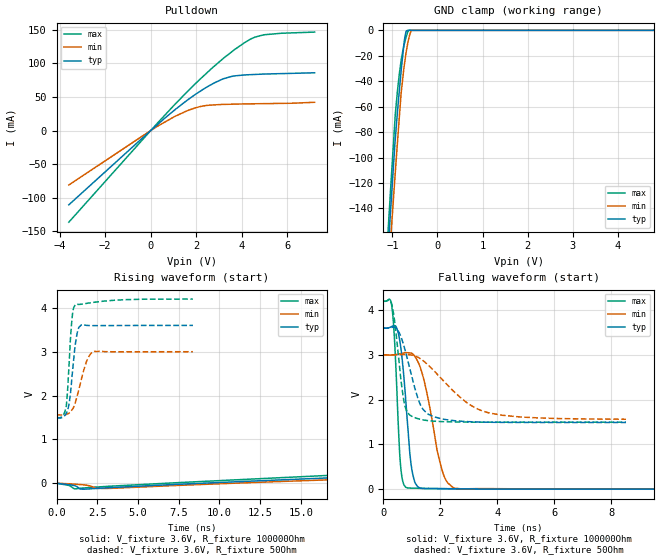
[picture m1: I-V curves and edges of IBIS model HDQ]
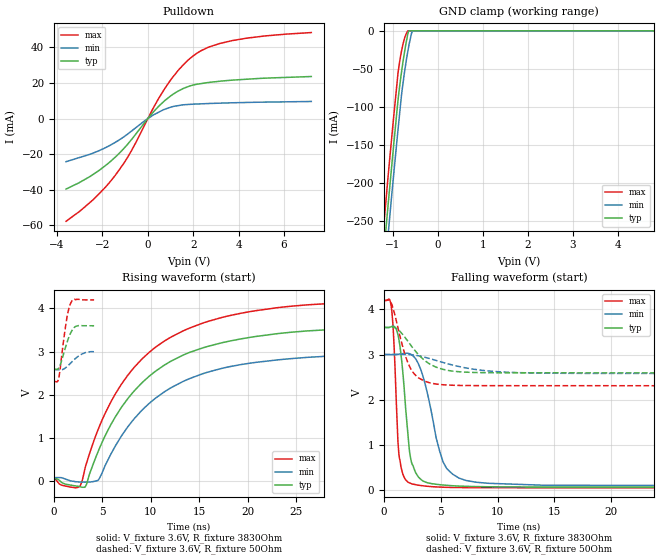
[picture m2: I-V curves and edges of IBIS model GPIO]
|Texas Instruments Incorporated
|Single-Cell Li-Ion and Li-Pol Battery Gas Gauge IC for Portable Applications
|   (bqJunior)
| Marketing part#   Digital Voltage Range   Package-type   #pins
| BQ27000DRKR   2.6 to 4.5V   VSON   10
| BQ27000DRKRG4   2.6 to 4.5V   VSON   10
[IBIS Ver]   3.2
[File name]   bq27000.ibs
|SIMDE Ver   V2.0 - 201002 - RHL4 - Build 372
[File Rev]   1.5
[Date]   08/18/2010
[Source]
|   Texas Instruments Incorporated.
|   Analog-eLab Design Center, HPA
|   12500 TI Blvd
|   Dallas, TX -75243
|   e-mail: elab_ibis@list.ti.com
| Model generated from simulations in TISPICE
[Notes]   Revision History:
|   Rev 1.0: 06/16/2010
|   - Initial version of the model
|   - Model names with a trailing 3p3pv contains the model for
|   3.3V [2.6V and 4.2V]. Model names with trailing 4p4v contains
|   the model for 4.4V [4.3V and 4.5V] operation.Model names with
|   trailing 3p5v contains the model for 3.55V [2.6 and 4.5V]
|   operation.
|   Rev 1.1: 07/02/2010
|   - Model generated from simulations in TISPICE
|   - Model matched to SPICE simulation
|   - Updated the ibis file with data sheet title and package
|   details
|   - While calculating R_pkg, L_pkg and C_pkg ignored values
|   corresponding to power and ground pins
|   - Added package details beside [Package]
|   - Updated the buffer ibis models with correct voltage ranges
|   - Model names with a trailing 3p6v contains the model for
|   3.6V [3.0V and 4.2V].
|   - C_comp although listed in numerical order of value are obtained
|   from varying PVT conditions. For PVT conditions for each specific
|   value refer the buffer description under respective [Model]. IBIS
|   model user is responsible for using appropriate C_comp to simulate
|   for Signal Integrity.
|*   EXCEPTION:   *
|*   - input_mode1_3p6v,input_mode2_3p6v and input_mode4_3p6v there will*
|*   be a leakage current in the clamp I-V table because of the   *
|*   pulldown on pad.   *
|   Rev 1.2: 07/13/2010
|   - IBIS models generated with updated temperature range(-20/25/70)
|   - Updated the package details.
|   - Removed input IBIS models with weak pulldown to pad.
|*   EXCEPTION:   *
|*   - input_mode4_3p6v there will be a leakage current in the clamp I-V*
|*   table because of the pulldown on pad.   *
|   Rev 1.3: 07/28/2010
|   - Changed open_drain model to io_open_drain
|   - Updated the package details.
|   - Corrected over voltage entries for INPUT buffer power clamp and
|   ground clamp tables.
|*   EXCEPTION:   *
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[Disclaimer]
| This model is designed as an aid for customers of Texas Instruments.
| TI and its licensors and suppliers make no warranties, either expressed
| or implied, with respect to this  model, including the warranties of
| merchantability or fitness for a particular purpose. The model is
| provided solely on an "as is" basis. The entire risk as to its quality
| and performance is with the customer.
[Copyright]
|(C) Copyright 2010 Texas Instruments Incorporated.All rights reserved.
|   BQ27000
[Component]   BQ27000
[Manufacturer]  TI
[Package]   | 10 VSON - DRK package
|   typ   min   max
R_pkg   0.049698   0.04509   0.0584
L_pkg   0.910128nH   0.82212nH   1.09342nH
C_pkg   0.140814pF   0.12909pF   0.15381pF
[Pin]  signal_name model_name   R_pin   L_pin   C_pin
1   RBI   TERM   0.05840   1.09342nH   0.14472pF
2   VCC   POWER   0.05274   0.97555nH   0.15314pF
3   VSS   GND   0.04627   0.84523nH   0.14454pF
4   D/C   TERM   0.04509   0.82212nH   0.14082pF
5   HDQ   HDQ   0.04667   0.85344nH   0.12909pF
6   BAT   TERM   0.04824   0.87702nH   0.13320pF
7   SRN   TERM   0.04798   0.87136nH   0.14749pF
8   SRP   TERM   0.05430   1.00150nH   0.15381pF
9   GPIO   GPIO   0.04775   0.86672nH   0.14403pF
10   PGM   TERM   0.04915   0.89544nH   0.13335pF
11   VSS   GND   0.00002   0.05199nH   0.50818pF
|   TERM Model
[Model] TERM
Model_type Terminator
C_comp   0   0   0
| variable   typ   min   max
[Voltage Range]   3.6   3   4.2
[POWER Clamp Reference]  3.6   3   4.2
[GND Clamp Reference]   0.0V   0.0V   0.0V
|Operating Temperature
[Temperature Range]   25   70   -20
| Models and submodels in the file (3): HDQ (I/O_open_drain), GPIO (I/O_open_drain), TERM (Terminator)
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|   HDQ Model
[Model]   HDQ
Model_type   I/O_open_drain
Polarity   Inverting
Enable   Active-Low
Vinl = 0.7
Vinh = 1.5
Vmeas = 1.8
Vref = 3.6
Cref = 5pF
Rref = 100000
|   typ   min   max
|   (nom PVT)   (Fast PVT)   (Slow PVT)
|Average
C_comp   2.068e-12   1.732e-12   2.876e-12
|OFF state: BUFFER in HIGH IMPEDANCE
|C_comp   1.649e-12   1.632e-12   1.682e-12
|ON state : BUFFER OUTPUT TURNED LOW
|C_comp   2.487e-12   1.832e-12   4.071e-12
[Voltage Range]   3.6   3   4.2
|Ambient Temperature   25   70   -20
|Junction Temperature
[Temperature Range]   25   70   -20
[Pullup Reference]   3.6   3   4.2
[Pulldown Reference]   0   0   0
[Power Clamp Reference]   3.6   3   4.2
[GND Clamp Reference]   0   0   0
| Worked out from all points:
|   slope of the pulldown table from 0 to 0.54 V, typ, clamps not added: 33.7 ohm
|   GND clamp passes 1 mA (typ) near -0.70 V on its own axis
|   falling waveform, V_fixture 3.6V, R_fixture 100000Ohm: 20-80 % time 279ps typ, 549ps min, 180ps max; typ from 3.6 V to 0.001 V
|   rising waveform, V_fixture 3.6V, R_fixture 100000Ohm: 20-80 % time 225ns typ, 230ns min, 223ns max; typ from 0.001 V to 3.6 V
|   falling waveform, V_fixture 3.6V, R_fixture 50Ohm: 20-80 % time 551ps typ, 1.46ns min, 291ps max; typ from 3.6 V to 1.49 V
|   rising waveform, V_fixture 3.6V, R_fixture 50Ohm: 20-80 % time 350ps typ, 624ps min, 265ps max; typ from 1.49 V to 3.6 V
[Pulldown]
|   Voltage   I(typ)   I(min)   I(max)
-3.6V     -110.5mA   -81.05mA   -136.3mA
0V        0A         0A         0A
1.035V    30.07mA    20.52mA    37.86mA
1.674V    46.81mA    30.34mA    59.98mA
2.223V    59.47mA    35.97mA    78.03mA
2.794V    70.82mA    38.11mA    95.68mA
3.146V    76.31mA    38.77mA    106mA
3.683V    81.19mA    39.21mA    120.3mA
4.38V     83.04mA    39.68mA    135.8mA
4.582V    83.35mA    39.77mA    138.9mA
4.968V    83.94mA    39.95mA    142.3mA
7.2V      85.83mA    41.98mA    146.3mA
[GND Clamp]
|   Voltage   I(typ)   I(min)   I(max)
-3.6V     -1.773A    -1.701A    -1.839A
-1.143V   -199.5mA   -220.7mA   -185.7mA
-1.055V   -149.5mA   -172.9mA   -133.3mA
-1.023V   -131.9mA   -155.7mA   -115.1mA
-937.2mV  -85.84mA   -112.2mA   -66.69mA
-891mV    -65.5mA    -89.46mA   -48.68mA
-807mV    -32.17mA   -49.63mA   -23.81mA
-730.8mV  -7.013mA   -26.14mA   -10.08mA
-694.8mV  -545.6uA   -17.14mA   -5.281mA
-660mV    0A         -10.17mA   -1.416mA
-576mV    0A         0A         0A
7.2V      0A         0A         0A
[POWER Clamp]
|   Voltage   I(typ)   I(min)   I(max)
-3.6V     0A         0A         0A
7.2V      0A         0A         0A
[Ramp]
R_load = 100000
|   typ   min   max
dV/dt_r   2.15645/2.25529e-07   1.79638/2.30137e-07   2.51628/2.23208e-07
dV/dt_f   2.15929/2.80954e-10   1.79917/5.49564e-10   2.51932/1.84623e-10
[Falling Waveform]
V_fixture = 3.6V
V_fixture_min = 3V
V_fixture_max = 4.2V
R_fixture = 100000Ohm
|   Time   V(typ)   V(min)   V(max)
0s        3.6V       3V         4.2V
300ps     3.638V     2.999V     4.067V
400ps     3.65V      3.005V     3.229V
600ps     3.218V     3.028V     550.5mV
875ps     1.242V     3.048V     25.56mV
1ns       440.2mV    3.037V     23.89mV
1.2ns     59.77mV    2.864V     21.87mV
2.1ns     14.42mV    346.7mV    8.533mV
2.55ns    9.999mV    16.73mV    6.274mV
40ns      1.209mV    1.432mV    1.127mV
[Rising Waveform]
V_fixture = 3.6V
V_fixture_min = 3V
V_fixture_max = 4.2V
R_fixture = 100000Ohm
|   Time   V(typ)   V(min)   V(max)
0s        1.177mV    1.371mV    1.116mV
1.7ns     -132.9mV   -36.04mV   -105.1mV
3.25ns    -98.77mV   -115.3mV   -66.45mV
82ns      1.089V     882.5mV    1.301V
167.2ns   2.074V     1.696V     2.456V
241.1ns   2.651V     2.18V      3.123V
325.4ns   3.063V     2.528V     3.594V
423.2ns   3.326V     2.756V     3.894V
548.5ns   3.486V     2.896V     4.074V
1us       3.595V     2.995V     4.195V
[Falling Waveform]
V_fixture = 3.6V
V_fixture_min = 3V
V_fixture_max = 4.2V
R_fixture = 50Ohm
|   Time   V(typ)   V(min)   V(max)
0s        3.6V       3V         4.2V
300ps     3.616V     3.001V     4.114V
500ps     3.559V     3.006V     3.15V
725ps     3.19V      3.009V     1.953V
1.05ns    2.391V     2.991V     1.612V
1.3ns     1.886V     2.914V     1.561V
1.6ns     1.667V     2.757V     1.53V
2.9ns     1.512V     1.949V     1.5V
3.6ns     1.497V     1.724V     1.499V
8.525ns   1.491V     1.563V     1.498V
[Rising Waveform]
V_fixture = 3.6V
V_fixture_min = 3V
V_fixture_max = 4.2V
R_fixture = 50Ohm
|   Time   V(typ)   V(min)   V(max)
0s        1.49V      1.56V      1.498V
375ps     1.504V     1.556V     1.538V
600ps     1.599V     1.57V      1.768V
775ps     1.828V     1.603V     2.736V
925ps     2.322V     1.661V     3.641V
1.15ns    3.151V     1.837V     4.069V
1.4ns     3.567V     2.179V     4.078V
1.825ns   3.601V     2.759V     4.1V
2.25ns    3.594V     3V         4.123V
8.375ns   3.599V     2.999V     4.199V
|   GPIO Model
[Model]   GPIO
Model_type   I/O_open_drain
Polarity   Non-Inverting
Enable   Active-Low
Vinl = 0.7
Vinh = 1.5
Vmeas = 1.8
Vref = 3.6
Cref = 5pF
Rref = 3830
|   typ   min   max
|   (nom PVT)   (Fast PVT)   (Slow PVT)
|Average
C_comp   3.532e-12   2.936e-12   3.781e-12
|ON state : BUFFER OUTPUT TURNED LOW
|C_comp   5.491e-12   4.260e-12   6.024e-12
|OFF state: BUFFER in HIGH IMPEDANCE
|C_comp   1.574e-12   1.613e-12   1.538e-12
[Voltage Range]   3.6   3   4.2
|Ambient Temperature   25   70   -20
|Junction Temperature
[Temperature Range]   25   70   -20
[Pullup Reference]   3.6   3   4.2
[Pulldown Reference]   0   0   0
[Power Clamp Reference]   3.6   3   4.2
[GND Clamp Reference]   0   0   0
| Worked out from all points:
|   slope of the pulldown table from 0 to 0.54 V, typ, clamps not added: 70.8 ohm
|   GND clamp passes 1 mA (typ) near -0.65 V on its own axis
|   falling waveform, V_fixture 3.6V, R_fixture 3830Ohm: 20-80 % time 756ps typ, 1.59ns min, 432ps max; typ from 3.6 V to 0.059 V
|   rising waveform, V_fixture 3.6V, R_fixture 3830Ohm: 20-80 % time 8.23ns typ, 8.29ns min, 8.21ns max; typ from 0.059 V to 3.58 V
|   falling waveform, V_fixture 3.6V, R_fixture 50Ohm: 20-80 % time 2.2ns typ, 4.24ns min, 1.34ns max; typ from 3.6 V to 2.59 V
|   rising waveform, V_fixture 3.6V, R_fixture 50Ohm: 20-80 % time 859ps typ, 1.26ns min, 680ps max; typ from 2.59 V to 3.6 V
[Pulldown]
|   Voltage   I(typ)   I(min)   I(max)
-3.6V     -39.56mA   -24.2mA    -57.68mA
-2.407V   -31.35mA   -19.38mA   -45.57mA
-1.441V   -21.75mA   -13.42mA   -31.99mA
-748.2mV  -12.24mA   -7.324mA   -18.68mA
230.4mV   3.507mA    1.925mA    5.685mA
755.4mV   10.18mA    5.247mA    17.04mA
1.369V    15.62mA    7.331mA    27.52mA
1.986V    18.78mA    8.072mA    35.07mA
2.696V    20.29mA    8.456mA    40.19mA
3.712V    21.57mA    8.853mA    43.76mA
5.165V    22.69mA    9.232mA    46.39mA
7.2V      23.61mA    9.596mA    48.28mA
[GND Clamp]
|   Voltage   I(typ)   I(min)   I(max)
-3.6V     -2.014A    -2.032A    -2.001A
-1.202V   -291.3mA   -330.8mA   -254.4mA
-1.128V   -242mA     -281.4mA   -204.4mA
-1.094V   -219.9mA   -259.4mA   -182.2mA
-1.023V   -174.6mA   -213.1mA   -137.2mA
-886.8mV  -90.4mA    -129.4mA   -54.74mA
-810mV    -54.05mA   -84.3mA    -26.45mA
-777.6mV  -40.65mA   -69.31mA   -17.48mA
-669.6mV  -3.959mA   -27.01mA   0A
-642mV    0A         -17.85mA   0A
-563.4mV  0A         0A         0A
7.2V      0A         0A         0A
[POWER Clamp]
|   Voltage   I(typ)   I(min)   I(max)
-3.6V     0A         0A         0A
7.2V      0A         0A         0A
[Ramp]
R_load = 3830
|   typ   min   max
dV/dt_r   2.11323/8.20281e-09   1.73333/8.26764e-09   2.48438/8.20667e-09
dV/dt_f   2.12482/7.53323e-10   1.74786/1.58248e-09   2.49431/4.30495e-10
[Falling Waveform]
V_fixture = 3.6V
V_fixture_min = 3V
V_fixture_max = 4.2V
R_fixture = 3830Ohm
|   Time   V(typ)   V(min)   V(max)
0s        3.6V       3V         4.2V
700ps     3.625V     3V         3.933V
900ps     3.624V     3V         3.118V
1.25ns    3.414V     3.007V     979mV
1.625ns   2.689V     3.019V     376.1mV
2.2ns     965.7mV    3.022V     157.1mV
3.375ns   204.3mV    2.563V     90.38mV
5.225ns   105.6mV    605.2mV    56.79mV
7.15ns    77.23mV    211.6mV    48.44mV
40ns      58.64mV    86.9mV     42.82mV
[Rising Waveform]
V_fixture = 3.6V
V_fixture_min = 3V
V_fixture_max = 4.2V
R_fixture = 3830Ohm
|   Time   V(typ)   V(min)   V(max)
0s        58.54mV    86.72mV    42.68mV
2.5ns     -114.2mV   -12.15mV   -138mV
2.825ns   -131.2mV   -15.36mV   -46.34mV
3.2ns     -136.1mV   -17mV      285.7mV
4.575ns   695.1mV    28.15mV    1.204V
7.025ns   1.73V      1.069V     2.266V
9.825ns   2.43V      1.802V     2.983V
13.33ns   2.92V      2.311V     3.479V
23.1ns    3.417V     2.81V      4.018V
40ns      3.581V     2.976V     4.183V
[Falling Waveform]
V_fixture = 3.6V
V_fixture_min = 3V
V_fixture_max = 4.2V
R_fixture = 50Ohm
|   Time   V(typ)   V(min)   V(max)
0s        3.6V       3V         4.2V
425ps     3.6V       3V         4.209V
675ps     3.606V     3V         4.118V
1.775ns   3.405V     3.002V     3.056V
2.35ns    3.21V      2.996V     2.686V
3ns       3.007V     2.973V     2.49V
3.925ns   2.806V     2.917V     2.38V
5.925ns   2.636V     2.774V     2.32V
10.03ns   2.596V     2.619V     2.309V
25ns      2.594V     2.58V      2.308V
[Rising Waveform]
V_fixture = 3.6V
V_fixture_min = 3V
V_fixture_max = 4.2V
R_fixture = 50Ohm
|   Time   V(typ)   V(min)   V(max)
0s        2.594V     2.58V      2.308V
350ps     2.593V     2.58V      2.304V
525ps     2.625V     2.579V     2.408V
1.325ns   3.188V     2.647V     3.751V
1.525ns   3.319V     2.69V      3.972V
1.75ns    3.437V     2.74V      4.125V
2ns       3.531V     2.795V     4.207V
2.35ns    3.591V     2.863V     4.208V
3.225ns   3.599V     2.975V     4.196V
4.15ns    3.598V     2.998V     4.196V
